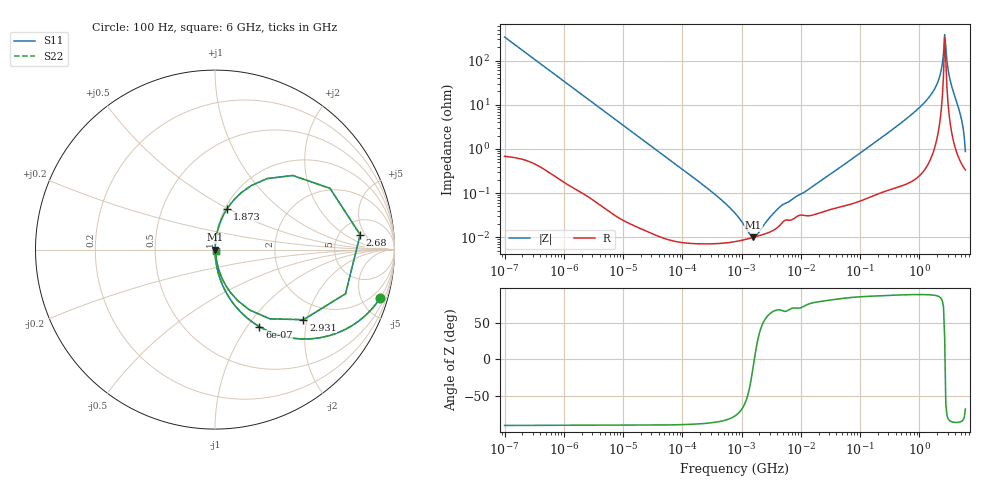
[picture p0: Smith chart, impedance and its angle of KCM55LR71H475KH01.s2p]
!Murata Part Number: KCM55LR71H475KH01
!These Parameters are Measured in Series Mode Connection
!Data Generated on Mar 13, 2026
!  o--ll--o
!Port1  Port2
!  o------o
!Operation Temp=25[degC], DC Bias Voltage=0[V]
!Freq. Start=100[Hz] Stop=6[GHz] 401[Steps]
# Hz S RI R 50
!Freq.(Hz) S11(Real) S11(Imag) S21(Real) S21(Imag) S12(Real) S12(Imag) S22(Real) S22(Imag)
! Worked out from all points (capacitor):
!   401 points, 100 Hz to 6 GHz, reference 50 ohm
!   read as one part in series: C = 4.66 uF near 109 Hz
!   lowest |Z| = 10.1 mohm at 1.586 MHz (marker M1)
!   series resonance near 1.642 MHz, so ESL is about 2 nH
!   S11 on the Smith chart (normalised r, x): 100 Hz: 1.01, -6.83; 600 Hz: 1.01, -1.14; 1.873 GHz: 1.02, +0.50; 2.68 GHz: 7.80, +3.82; 2.931 GHz: 1.48, -1.91; 6 GHz: 1.01, -0.02
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100  0.9206 -0.2693  0.0794 0.2693  0.0794 0.2693  0.9206 -0.2693
280  0.5986 -0.4881  0.4014 0.4881  0.4014 0.4881  0.5986 -0.4881
600  0.2479 -0.4294  0.7521 0.4294  0.7521 0.4294  0.2479 -0.4294
2008  0.0295 -0.1663  0.9705 0.1663  0.9705 0.1663  0.0295 -0.1663
40335  0.000179 -0.00863  0.9998 0.00863  0.9998 0.00863  0.000179 -0.00863
316350  7.22e-05 -0.00106  0.9999 0.00106  0.9999 0.00106  7.22e-05 -0.00106
774597  7.97e-05 -0.000342  0.9999 0.000342  0.9999 0.000342  7.97e-05 -0.000342
1585629  9.96e-05 -1.38e-05  0.9999 1.38e-05  0.9999 1.38e-05  9.96e-05 -1.38e-05
4440638  0.000187 0.00045  0.9998 -0.00045  0.9998 -0.00045  0.000187 0.00045
1.555665e7  0.000318 0.00135  0.9997 -0.00135  0.9997 -0.00135  0.000318 0.00135
3.124326e8  0.00177 0.0243  0.9982 -0.0243  0.9982 -0.0243  0.00177 0.0243
1.046602e9  0.0107 0.0898  0.9893 -0.0898  0.9893 -0.0898  0.0107 0.0898
1.873145e9  0.068 0.2281  0.932 -0.2281  0.932 -0.2281  0.068 0.2281
2.142435e9  0.1458 0.3166  0.8542 -0.3166  0.8542 -0.3166  0.1458 0.3166
2.34314e9  0.2898 0.3956  0.7102 -0.3956  0.7102 -0.3956  0.2898 0.3956
2.450438e9  0.4334 0.4129  0.5666 -0.4129  0.5666 -0.4129  0.4334 0.4129
2.679998e9  0.8087 0.083  0.1913 -0.083  0.1913 -0.083  0.8087 0.083
2.931063e9  0.493 -0.3905  0.507 0.3905  0.507 0.3905  0.493 -0.3905
3.205649e9  0.1926 -0.3364  0.8074 0.3364  0.8074 0.3364  0.1926 -0.3364
3.666503e9  0.0603 -0.2005  0.9397 0.2005  0.9397 0.2005  0.0603 -0.2005
5.016141e9  0.00789 -0.054  0.9921 0.054  0.9921 0.054  0.00789 -0.054
6e9  0.0034 -0.00803  0.9966 0.00803  0.9966 0.00803  0.0034 -0.00803
